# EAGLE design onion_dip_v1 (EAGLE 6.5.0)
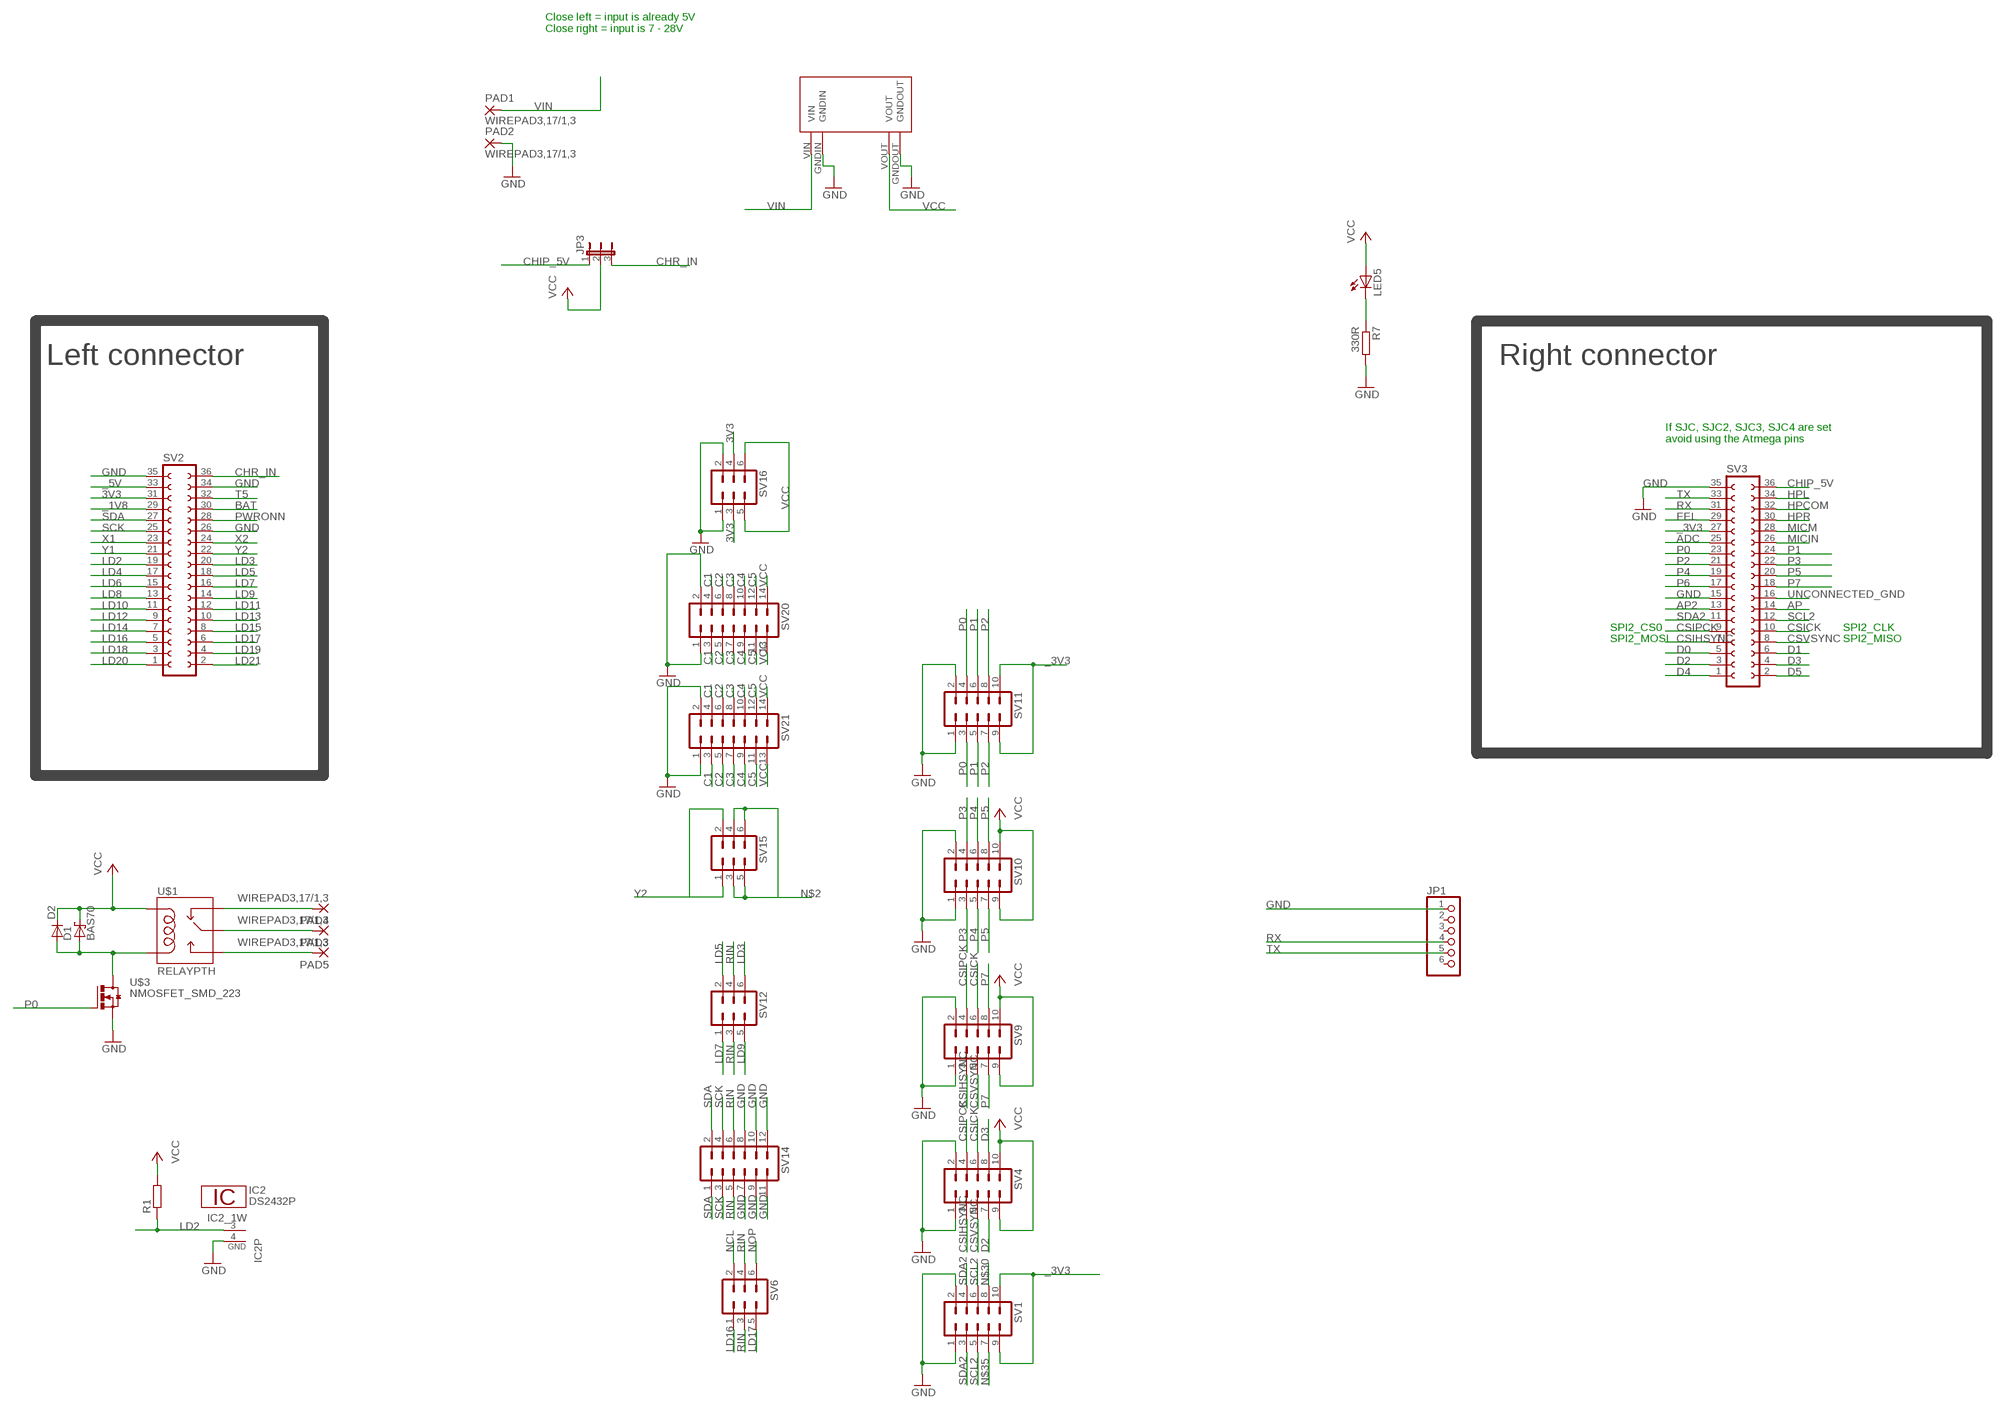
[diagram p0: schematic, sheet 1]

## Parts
D1  BAS70  [SOT23]
D2  DIODE-SMB  [SMB]
IC2  DS2432P  [TSOC6]
JP1  PINHD-1X6  [1X06]
JP3  JP2E  [JP2]
LED5  LEDCHIP-LED0805  [CHIP-LED0805]
PAD1  WIREPAD3,17/1,3  [3,17/1,3]
PAD2  WIREPAD3,17/1,3  [3,17/1,3]
PAD3  WIREPAD3,17/1,3  [3,17/1,3]
PAD4  WIREPAD3,17/1,3  [3,17/1,3]
PAD5  WIREPAD3,17/1,3  [3,17/1,3]
R1  R-EU_R0805  [R0805]
R7  330R  R-EU_R0805  [R0805]
SV1  MA05-2  [MA05-2]
SV2  FE18-2  [FE18-2]
SV3  FE18-2  [FE18-2]
SV4  MA05-2  [MA05-2]
SV6  MA03-2  [MA03-2]
SV9  MA05-2  [MA05-2]
SV10  MA05-2  [MA05-2]
SV11  MA05-2  [MA05-2]
SV12  MA03-2  [MA03-2]
SV14  MA06-2  [MA06-2]
SV15  MA03-2  [MA03-2]
SV16  MA03-2  [MA03-2]
SV20  MA07-2  [MA07-2]
SV21  MA07-2  [MA07-2]
U$1  RELAYPTH  [SRD-05VDC-SL-C]
U$3  NMOSFET_SMD_223  [SOT223]
U$9  MP1584EN  [MP1584EN]

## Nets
3V3: SV2.31 SV16.3 SV16.4
_1V8: SV2.29
_3V3: SV1.9 SV1.10 SV3.27 SV11.9 SV11.10
_5V: SV2.33
ADC: SV3.25
AP: SV3.14
AP2: SV3.13
BAT: SV2.30
C1: SV20.3 SV20.4 SV21.3 SV21.4
C2: SV20.5 SV20.6 SV21.5 SV21.6
C3: SV20.7 SV20.8 SV21.7 SV21.8
C4: SV20.9 SV20.10 SV21.9 SV21.10
C5: SV20.11 SV20.12 SV21.11 SV21.12
CHIP_5V: JP3.1 SV3.36
CHR_IN: JP3.3 SV2.36
CSICK: SV3.10 SV4.6 SV9.6
CSIHSYNC: SV3.7 SV4.3 SV9.3
CSIPCK: SV3.9 SV4.4 SV9.4
CSVSYNC: SV3.8 SV4.5 SV9.5
D0: SV3.5
D1: SV3.6
D2: SV3.3 SV4.7
D3: SV3.4 SV4.8
D4: SV3.1
D5: SV3.2
FEL: SV3.29
GND: IC2.4(GND) JP1.1 PAD2.1(P) R7.2 SV1.1 SV1.2 SV2.26 SV2.34 SV2.35 SV3.15 SV3.35 SV4.1 SV4.2 SV9.1 SV9.2 SV10.1 SV10.2 SV11.1 SV11.2 SV14.7 SV14.8 SV14.9 SV14.10 SV14.11 SV14.12 SV16.1 SV16.2 SV20.1 SV20.2 SV21.1 SV21.2 U$3.3(S) U$9.GNDIN U$9.GNDOUT
HPCOM: SV3.32
HPL: SV3.34
HPR: SV3.30
LD2: IC2.3(1W) R1.1 SV2.19
LD3: SV2.20 SV12.6
LD4: SV2.17
LD5: SV2.18 SV12.2
LD6: SV2.15
LD7: SV2.16 SV12.1
LD8: SV2.13
LD9: SV2.14 SV12.5
LD10: SV2.11
LD11: SV2.12
LD12: SV2.9
LD13: SV2.10
LD14: SV2.7
LD15: SV2.8
LD16: SV2.5 SV6.1
LD17: SV2.6 SV6.5
LD18: SV2.3
LD19: SV2.4
LD20: SV2.1
LD21: SV2.2
MICIN: SV3.26
MICM: SV3.28
N$1: D1.1(A) D2.A U$1.COIL0 U$3.2(D) U$3.4(D)
N$2: SV15.3 SV15.4 SV15.5 SV15.6
N$29: LED5.C R7.1
N$30: SV1.8
N$35: SV1.7
NCL: PAD4.1(P) SV6.2 U$1.SWCLOSED(SWCLOSE)
NOP: PAD5.1(P) SV6.6 U$1.SWOPEN
P0: SV3.23 SV11.3 SV11.4 U$3.1(G)
P1: SV3.24 SV11.5 SV11.6
P2: SV3.21 SV11.7 SV11.8
P3: SV3.22 SV10.3 SV10.4
P4: SV3.19 SV10.5 SV10.6
P5: SV3.20 SV10.7 SV10.8
P6: SV3.17
P7: SV3.18 SV9.7 SV9.8
PWRONN: SV2.28
RIN: PAD3.1(P) SV6.3 SV6.4 SV12.3 SV12.4 SV14.5 SV14.6 U$1.SWCOMMON
RX: JP1.4 SV3.31
SCK: SV2.25 SV14.3 SV14.4
SCL2: SV1.5 SV1.6 SV3.12
SDA: SV2.27 SV14.1 SV14.2
SDA2: SV1.3 SV1.4 SV3.11
T5: SV2.32
TX: JP1.5 SV3.33
UNCONNECTED_GND: SV3.16
VCC: D1.3(C) D2.C JP3.2 LED5.A R1.2 SV4.9 SV4.10 SV9.9 SV9.10 SV10.9 SV10.10 SV16.5 SV16.6 SV20.13 SV20.14 SV21.13 SV21.14 U$1.COIL1 U$9.VOUT
VIN: PAD1.1(P) U$9.VIN
X1: SV2.23
X2: SV2.24
Y1: SV2.21
Y2: SV2.22 SV15.1 SV15.2
Unconnected: JP1.2 JP1.3 JP1.6

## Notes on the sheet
- Close left = input is already 5V
  Close right = input is 7 - 28V
- Left connector | Right connector
- If SJC, SJC2, SJC3, SJC4 are set 
  avoid using the Atmega pins
- SPI2_CS0 | SPI2_CLK
- SPI2_MOSI | SPI2_MISO

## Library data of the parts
D1 = diode:BAS70: Silicon Schottky Diodes
D2 = diode:DIODE-: DIODE
IC2 = 1wire:DS2432: 1024-Bit Protected EEPROM with SHA-1 Engine
JP1 = pinhead:PINHD-1X6: PIN HEADER
JP3 = jumper:JP2E: JUMPER
LED5 = led:LED: LED
PAD1-PAD5 = wirepad:WIREPAD: Wire PAD connect wire on PCB
R1 R7 = rcl:R-EU_: RESISTOR, European symbol
SV1 SV4 SV9-SV11 = con-lstb:MA05-2: PIN HEADER; OC_FARNELL: unknown; OC_NEWARK: unknown
SV2 SV3 = con-lsta:FE18-2: FEMALE HEADER; OC_FARNELL: unknown; OC_NEWARK: unknown
SV6 SV12 SV15 SV16 = con-lstb:MA03-2: PIN HEADER; OC_FARNELL: unknown; OC_NEWARK: unknown
SV14 = con-lstb:MA06-2: PIN HEADER; OC_FARNELL: unknown; OC_NEWARK: unknown
SV20 SV21 = con-lstb:MA07-2: PIN HEADER; OC_FARNELL: unknown; OC_NEWARK: unknown
U$1 = SRD-05VDC-SL-C:RELAY: SPDT relay (COM-00101)
U$3 = transistor-power:NMOSFET_SMD_223
U$9 = power_supply:MP1584EN

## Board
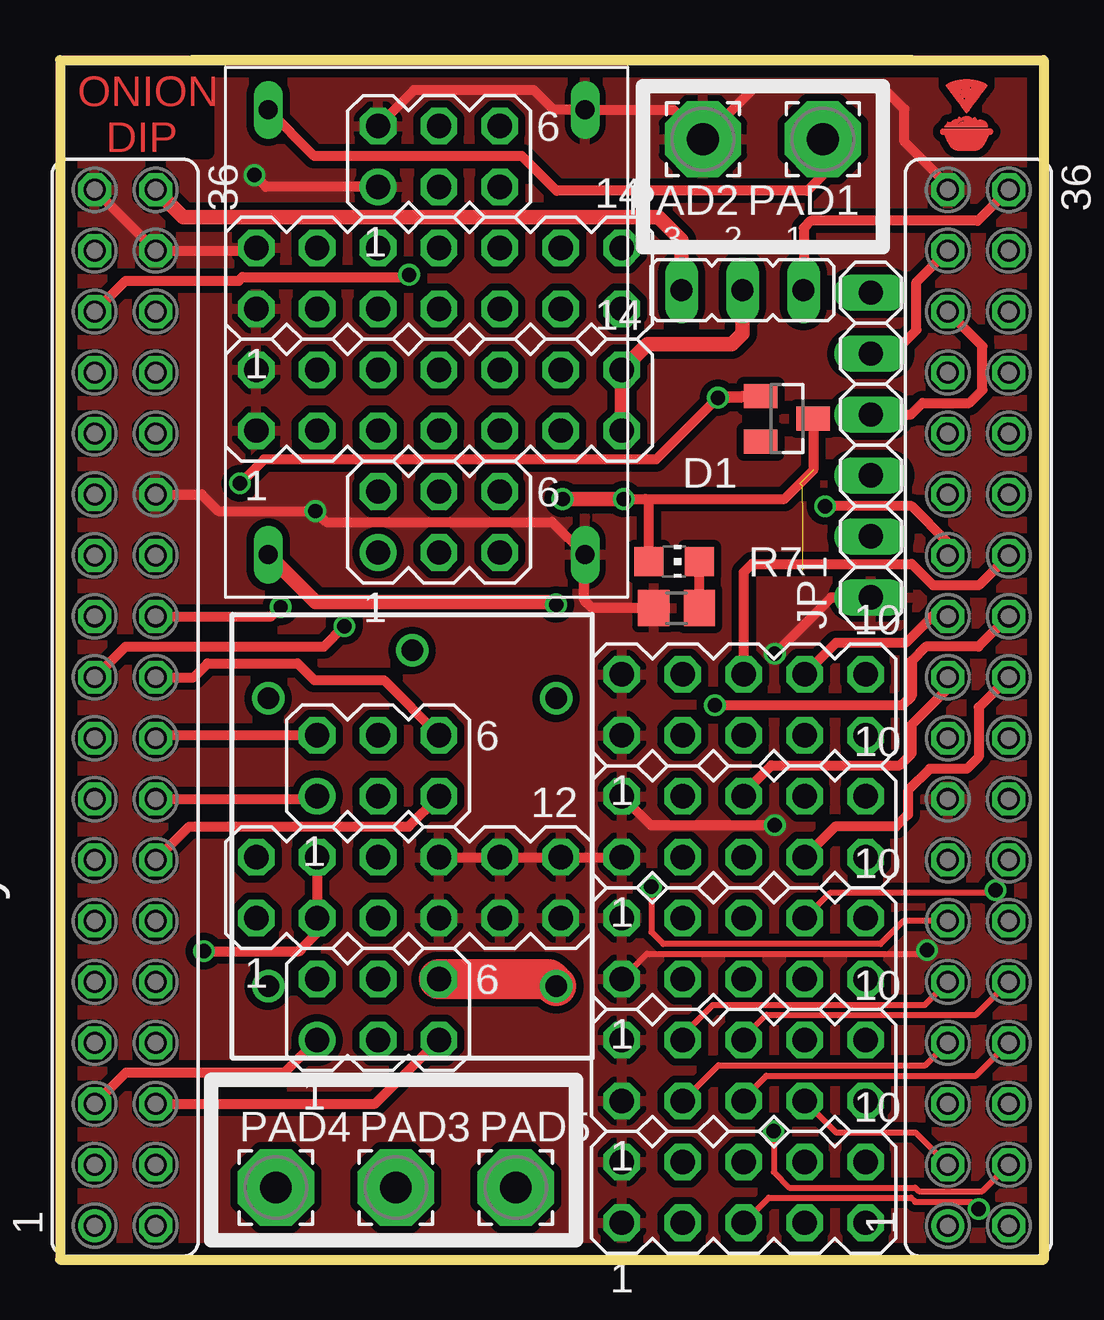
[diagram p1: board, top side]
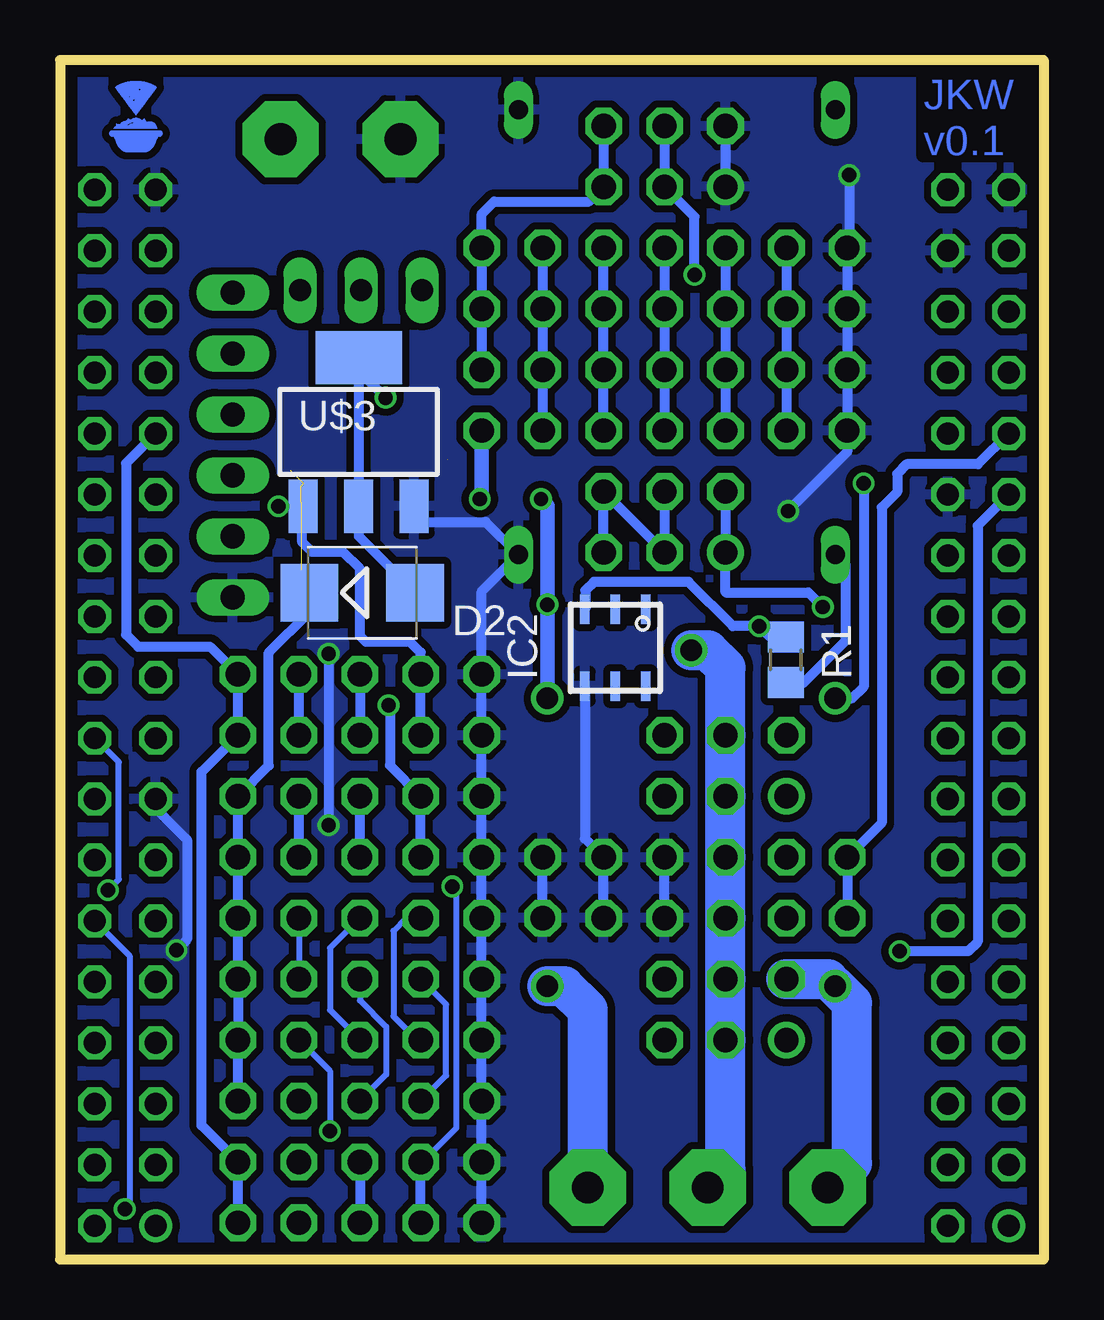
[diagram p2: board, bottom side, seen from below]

Size 41 x 50 mm. Coordinates in mm from the lower left corner, seen from the top.
Outline: 0,50 41,50 41,0 0,0 0,50
Copper layers (1*16): Top 0.035mm / dielectric 1.6mm / Bottom 0.035mm
Design rules "Elecrow_2-layer_PCB_eagle_rule": minimum track width 6mil, minimum drill 12mil, track to track 6mil, track to pad 6mil, pad to pad 6mil, via to via 8mil, smd to smd 0mil, copper to edge 20mil, drill to drill 10mil, minimum pad ring 6mil, minimum via ring 6mil, stop-mask expansion 0mil, vias tented up to drill 100mil, thermal gap 10mil

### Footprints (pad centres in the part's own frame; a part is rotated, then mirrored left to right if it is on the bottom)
SOT23 = smd 1 x 1.4: 1 -0.95,-1.1; 2 0.95,-1.1; 3 0,1.1
SMB = smd 2.4 x 2.4: A 2.2,0; C -2.2,0
TSOC6 = smd 0.406 x 1.219: 1 -1.27,-1.6; 2 0,-1.6; 3 1.27,-1.6; 4 1.27,1.6; 5 0,1.6; 6 -1.27,1.6
1X06 = drill 1.016 long: 1 -6.35,0; 2 -3.81,0; 3 -1.27,0; 4 1.27,0; 5 3.81,0; 6 6.35,0
JP2 = drill 0.914 long: 1 -2.54,0; 2 0,0; 3 2.54,0
CHIP-LED0805 = smd 1.2 x 1.2: A 0,-1.05; C 0,1.05
3,17/1,3 = drill 1.321 pad 3.175 octagon: 1 0,0
R0805 = smd 1.3 x 1.5: 1 -0.95,0; 2 0.95,0
MA05-2 = drill 1.016 octagon: 1 -5.08,-1.27; 2 -5.08,1.27; 3 -2.54,-1.27; 4 -2.54,1.27; 5 0,-1.27; 6 0,1.27; 7 2.54,-1.27; 8 2.54,1.27; 9 5.08,-1.27; 10 5.08,1.27
FE18-2 = drill 0.914: 1 -21.59,1.27 | drill 0.914 octagon: 2 -21.59,-1.27; 3 -19.05,1.27; 4 -19.05,-1.27; 5 -16.51,1.27; 6 -16.51,-1.27; 7 -13.97,1.27; 8 -13.97,-1.27; 9 -11.43,1.27; 10 -11.43,-1.27; 11 -8.89,1.27; 12 -8.89,-1.27; 13 -6.35,1.27; 14 -6.35,-1.27; 15 -3.81,1.27; 16 -3.81,-1.27; 17 -1.27,1.27; 18 -1.27,-1.27; 19 1.27,1.27; 20 1.27,-1.27; 21 3.81,1.27; 22 3.81,-1.27; 23 6.35,1.27; 24 6.35,-1.27; 25 8.89,1.27; 26 8.89,-1.27; 27 11.43,1.27; 28 11.43,-1.27; 29 13.97,1.27; 30 13.97,-1.27; 31 16.51,1.27; 32 16.51,-1.27; 33 19.05,1.27; 34 19.05,-1.27; 35 21.59,1.27; 36 21.59,-1.27
MA03-2 = drill 1.016: 1 -2.54,-1.27 | drill 1.016 octagon: 2 -2.54,1.27; 3 0,-1.27; 4 0,1.27; 5 2.54,-1.27; 6 2.54,1.27
MA06-2 = drill 1.016 octagon: 1 -6.35,-1.27; 2 -6.35,1.27; 3 -3.81,-1.27; 4 -3.81,1.27; 5 -1.27,-1.27; 6 -1.27,1.27; 7 1.27,-1.27; 8 1.27,1.27; 9 3.81,-1.27; 10 3.81,1.27; 11 6.35,-1.27; 12 6.35,1.27
MA07-2 = drill 1.016 octagon: 1 -7.62,-1.27; 2 -7.62,1.27; 3 -5.08,-1.27; 4 -5.08,1.27; 5 -2.54,-1.27; 6 -2.54,1.27; 7 0,-1.27; 8 0,1.27; 9 2.54,-1.27; 10 2.54,1.27; 11 5.08,-1.27; 12 5.08,1.27; 13 7.62,-1.27; 14 7.62,1.27
SRD-05VDC-SL-C = drill 0.9: COIL0 -5.39,-6.12; COIL1 -5.39,5.88; SWCLOSED 6.61,-6.12; SWCOMMON -7.39,-0.12; SWOPEN 6.61,5.88
SOT223 = smd 1.219 x 2.235: 1 -2.311,-3.099; 2 0,-3.099; 3 2.311,-3.099 | smd 3.6 x 2.2: 4 0,3.099
MP1584EN = drill 0.8 long: GNDIN 1.778,14.986; GNDOUT 20.32,14.986; VIN 1.778,1.778; VOUT 20.32,1.778

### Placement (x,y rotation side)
D1  30.3,35.05 270 top
D2  28.4,27.8 0 bottom
IC2  17.85,25.5 180 bottom
JP1  33.8,33.95 90 top
JP3  28.45,40.4 180 top
LED5  25.6,29.1 270 top
PAD1  31.8,46.7 180 top
PAD2  26.8,46.7 180 top
PAD3  14,3 0 top
PAD4  9,3 0 top
PAD5  19,3 0 top
R1  10.75,25 270 bottom
R7  25.7,27.15 180 top
SV1  28.5,2.8 0 top
SV2  2.72,23 90 top
SV3  38.28,23 90 top
SV4  28.5,7.88 0 top
SV6  13.26,10.42 0 top
SV9  28.5,12.96 0 top
SV10  28.5,18.04 0 top
SV11  28.5,23.12 0 top
SV12  13.26,20.58 0 top
SV14  14.53,15.5 0 top
SV15  15.8,30.74 0 top
SV16  15.8,45.98 0 top
SV20  15.8,40.9 0 top
SV21  15.8,35.82 0 top
U$1  14.8,18 270 top
U$2  LOGO  [LOGO]  36.54,46.02 0 top
U$3  28.55,34.5 0 bottom
U$5  LOGO  [LOGO]  39.09,46.1 0 bottom
U$9  6.9,49.7 270 top

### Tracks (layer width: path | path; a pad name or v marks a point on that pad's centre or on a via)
3V3  (via drill 0.6)
  Top 0.406: SV2.31 2.74,40.8 7.45,40.8 7.6,40.95 14.45,40.95 v14.55,41.05
  Bottom 0.406: v14.55,41.05 14.55,43.46 SV16.3 SV16.4
_3V3
  Bottom 0.406: SV1.9 SV1.10 35.1,5.59 35.1,20.33 SV11.9 SV11.10 34.74,25.55 37.75,25.55 38.25,26.05 38.25,33.19 SV3.27
C1
  Bottom 0.406: SV20.4 SV20.3 SV21.4 SV21.3
C2
  Bottom 0.406: SV20.6 SV20.5 SV21.6 SV21.5
C3
  Bottom 0.406: SV20.8 SV20.7 SV21.8 SV21.7
C4
  Bottom 0.406: SV21.9 SV21.10 SV20.9 SV20.10
C5
  Bottom 0.406: SV20.12 SV20.11 SV21.12 SV21.11
CHIP_5V
  Top 0.406: SV3.36 38.26,43.3 31.3,43.3 31,43 31,40.21 JP3.1
CHR_IN
  Top 0.61: SV2.36 5.13,43.45 24.95,43.45 25.91,42.49 JP3.3
CSICK
  Top 0.254: SV4.6 28.5,9.25 29.45,10.2 38.18,10.2 SV3.10
  Bottom 0.254: SV9.6 29.75,12.98 29.75,10.4 SV4.6
CSIHSYNC
  Top 0.254: SV4.3 27.45,8.1 36.08,8.1 SV3.7
  Bottom 0.254: SV9.3 24.9,10.63 24.9,7.67 SV4.3
CSIPCK
  Top 0.254: SV4.4 25.96,9.36 27.21,10.61 36.05,10.61 SV3.9
  Bottom 0.254: 26.42,14.23 SV9.4 26.57,14.23 27.1,13.7 27.1,10.14 26.11,9.15 SV4.4
CSVSYNC
  Top 0.254: SV3.8 38.18,7.66 29.44,7.66 28.5,6.72 SV4.5
  Bottom 0.254: SV9.5 28.5,10.8 27.4,9.7 27.4,7.71 SV4.5
D2
  Top 0.254: SV4.7 32.35,5.3 35.66,5.3 SV3.3
D3  (via drill 0.6)
  Top 0.254: v29.75,5.35 29.75,3.65 30.4,3 35.65,3 35.8,2.85 38.45,2.85 SV3.4
  Bottom 0.254: SV4.8 29.75,7.86 v29.75,5.35
GND  (via drill 0.6)
  Top 0.254: v36.15,12.9 35.99,12.74 24.47,12.74 SV9.1
  Top 0.406: SV3.35 37.01,44.79 35.2,46.6 35.2,47.95 34.35,48.8 28.9,48.8 PAD2.1 25.58,47.92 U$9.GNDIN 20.58,47.92 19.75,48.75 14.76,48.75 SV16.2 | SV2.35 SV2.34 8.06,42.05 SV20.2 | R7.2 22.2,27.15 21.85,27.5 21.85,29.34 U$9.GNDOUT 20.52,30.75 11.1,30.75 v10.65,31.2 6.6,31.2 5.91,31.89 SV2.26 | SV16.1 8.59,44.71 v8.1,45.2 | SV14.8 SV14.10 SV14.12 SV10.1 | JP1.1 32.15,27.6 v29.8,25.25 | v29.8,18.1 24.63,18.1 SV10.2
  Bottom 0.406: SV1.1 SV1.2 SV4.1 SV4.2 SV9.1 SV9.2 SV10.1 SV10.2 SV11.1 SV11.2 23.42,27.85 U$9.GNDOUT 23.26,30.75 25.7,30.75 26.24,31.29 U$3.3 | SV3.15 37.01,18.81 35.7,17.5 35.7,13.35 v36.15,12.9 | SV16.2 SV16.1 | v8.1,45.2 8.1,42.25 SV20.2 SV20.1 SV21.2 SV21.1 8.18,33.67 v10.65,31.2 | SV14.7 SV14.8 | SV14.9 SV14.10 19.12,17.55 IC2.4 | SV14.11 SV14.12 | v29.8,25.25 v29.8,18.1
  pour Top (isolate 0.305, rank 2): -0.07,0.25 40.88,0.25 41.01,10.57 41.01,50.01 0,50.01 0,10.47
  pour Bottom (isolate 0.305): 0,50 41.05,50 41.05,0.25 0.02,0.25 0.02,49.92
LD2  (via drill 0.6)
  Top 0.406: SV2.19 2.73,25.55 11,25.55 v11.85,26.4
  Bottom 0.406: IC2.3 19.1,27.12 19.1,27.9 18.75,28.25 14.8,28.25 12.95,26.4 v11.85,26.4 11.4,25.95 R1.1
LD3
  Top 0.406: SV2.20 5.57,24.27 6.15,24.85 9.9,24.85 10.6,24.15 13.5,24.15 SV12.6
LD5
  Top 0.406: SV12.2 4.11,21.85 SV2.18
LD7
  Top 0.406: SV2.16 10.6,19.19 SV12.1
LD9
  Top 0.406: SV2.14 5.39,18.05 14.54,18.05 SV12.5
LD16
  Top 0.406: SV2.5 2.76,7.8 9.37,7.8 SV6.1
LD17
  Top 0.406: SV2.6 13.14,6.49 SV6.5
N$1  (via drill 0.6)  (1 unrouted)
  Top 0.406: v7.5,32.35 8.5,33.35 24.85,33.35 v27.43,35.92 | v27.43,35.92 27.5,36 28.45,36 | 28.45,36 D1.1 | v27.43,35.92 28.38,35.92 28.45,36
  Bottom 0.406: v7.5,32.35 7.5,23.87 7.98,23.39 U$1.COIL0 | D2.A 28.55,30.15 U$3.2 U$3.4 28.55,37.05 v27.43,35.92
N$2
  Bottom 0.406: SV15.4 SV15.3 SV15.6 SV15.5
N$29
  Top 0.406: R7.1 LED5.C
NCL
  Bottom 0.406: 8.98,11.69 U$1.SWCLOSED
  Bottom 1.676: PAD4.1 7.98,4.02 7.98,10.69 U$1.SWCLOSED | SV6.2 8.98,11.69
NOP
  Top 1.676: SV6.6 20.38,11.69 U$1.SWOPEN
  Bottom 1.676: PAD5.1 19,10.41 19.98,11.39 U$1.SWOPEN
P0  (via drill 0.6)
  Top 0.406: SV3.23 37.01,29.89 35.5,31.4 v31.9,31.4
  Bottom 0.406: SV11.3 SV11.4 25.96,25.31 26.4,25.75 28.25,25.75 28.5,26 28.5,28.8 29.2,29.5 30.5,29.5 30.9,29.9 30.9,31.36 U$3.1 v31.9,31.4
P1
  Top 0.406: SV3.24 38.3,28.1 36.4,28.1 35.5,29 28.85,29 28.5,28.65 SV11.6
  Bottom 0.406: SV11.6 SV11.5
P2
  Top 0.406: SV3.21 36.36,26.81 35.25,25.7 32.35,25.7 SV11.8
  Bottom 0.406: SV11.7 SV11.8
P3  (via drill 0.6)
  Top 0.406: SV3.22 38.29,25.55 36.1,25.55 35.5,24.95 35.5,23.5 35.1,23.1 v27.3,23.1
  Bottom 0.406: v27.3,23.1 27.25,23.05 27.25,20.6 SV10.4 SV10.3
P4
  Top 0.406: SV10.6 28.5,19.45 29.65,20.6 35,20.6 35.5,21.1 35.5,22.3 37.01,23.81 SV3.19
  Bottom 0.406: SV10.5 SV10.6
P5
  Top 0.406: SV3.20 38.3,23.02 38.3,20.95 37.8,20.45 36.25,20.45 35.35,19.55 35.35,18.55 34.85,18.05 32.32,18.05 SV10.7
  Bottom 0.406: SV10.7 SV10.8
P7  (via drill 0.6)
  Top 0.254: v39,15.4 38.85,15.28 32.09,15.28 SV9.8
  Bottom 0.254: v39,15.4 38.55,15.85 38.55,20.73 SV3.18 | SV9.8 SV9.7
RIN
  Bottom 1.676: PAD3.1 13.26,3.74 SV6.3 SV6.4 SV14.5 SV14.6 SV12.3 SV12.4 13.26,24.67 13.98,25.39 U$1.SWCOMMON
RX
  Top 0.406: JP1.4 35.47,35.22 35.95,35.7 37.9,35.7 38.45,36.25 38.45,38.07 SV3.31
SCK  (via drill 0.6)
  Top 0.406: SV14.4 SV14.3 10.7,14.21 10.7,13.6 10.05,12.95 arc-90 9.95,12.85 v6,12.85
  Bottom 0.406: SV2.25 2.75,30.59 2.75,13.25 3.15,12.85 v6,12.85
SCL2  (via drill 0.6)
  Top 0.254: SV1.5 29.55,2.58 35.47,2.58 35.65,2.4 38,2.4 v38.3,2.1
  Bottom 0.254: SV3.12 38.1,12.66 38.1,2.3 v38.3,2.1
  Bottom 0.406: SV1.6 SV1.5
SDA
  Bottom 0.406: SV14.1 SV14.2 6.75,18.2 6.75,31.35 6.1,32 6.1,32.75 5.7,33.15 2.73,33.15 SV2.27
SDA2  (via drill 0.6)
  Top 0.254: v24.65,15.55 24.65,13.65 25.15,13.15 34.2,13.15 35.16,14.11 SV3.11
  Bottom 0.254: v24.65,15.55 24.47,15.45 24.47,5.48 25.88,4.07 SV1.4
  Bottom 0.406: SV1.3 SV1.4
TX
  Top 0.406: JP1.5 34.71,37.76 35.7,38.75 35.7,40.74 SV3.33
VCC  (via drill 0.6)  (5 unrouted)
  Top 0.406: 24.4,31.7 30.2,31.7 31.4,32.9 D1.3 | LED5.A 24.55,31.55 24.4,31.7 | v23.5,31.7 24.4,31.7
  Top 0.61: U$9.VOUT 10.66,27.4 20.58,27.4 v20.68,27.3 | SV21.13 SV21.14 24.48,38.15 28,38.15 28.45,38.6 JP3.2 | v20.95,31.7 v23.5,31.7
  Bottom 0.406: SV4.9 SV4.10 SV9.9 SV9.10 SV10.9 SV10.10 32.3,20.59 32.3,25.3 30.6,27 D2.C 30.95,28.75 | SV21.14 SV20.13 SV20.14 23.42,43.58 22.9,44.1 18.95,44.1 SV16.5 SV16.6 | 23.42,31.78 v23.5,31.7 | R1.2 10,24.05 8.25,25.8 8.25,28.95 U$9.VOUT
  Bottom 0.61: SV21.13 23.42,31.78 | U$1.COIL1 v20.68,27.3 20.68,31.43 v20.95,31.7
VIN
  Top 0.406: PAD1.1 31.8,45.2 31.15,44.55 20.7,44.55 19.25,46 10.6,46 U$9.VIN
Y2  (via drill 0.6)
  Top 0.406: SV2.22 8.81,26.81 v9.2,27.2
  Bottom 0.406: SV15.2 SV15.1 13.26,27.81 9.81,27.81 v9.2,27.2

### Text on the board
Top: ONION / DIP
Bottom: JKW / v0.1
tNames: not yet ordered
